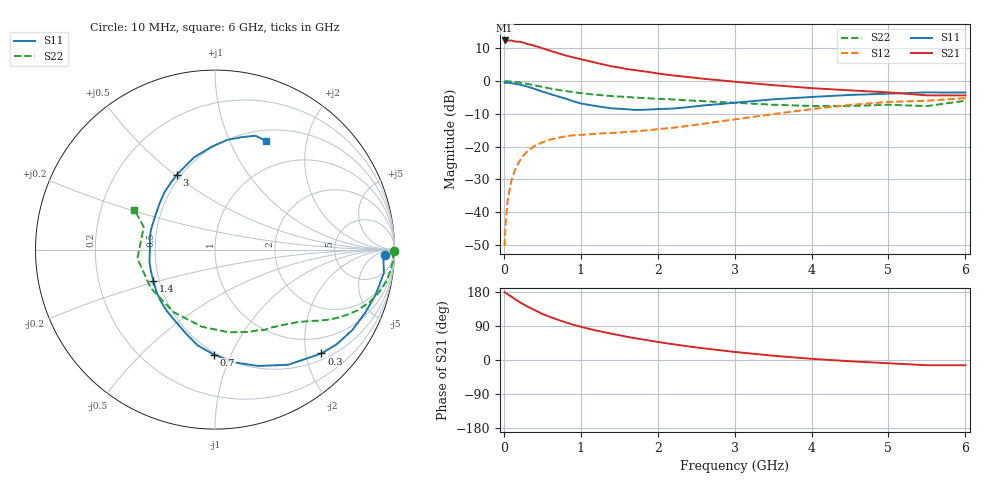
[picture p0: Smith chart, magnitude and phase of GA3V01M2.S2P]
! Infineon Technologies  Discrete & RF Semiconductors
! BF775
! Si NPN RF Bipolar Junction Transistor in SOT23
! VCE = 3 V  IC = 1.2 mA
! Common Emitter S-Parameters:  May  1996
# GHz  S  MA  R  50
!  f  S11  S21  S12  S22
! GHz  MAG  ANG  MAG  ANG  MAG  ANG  MAG  ANG
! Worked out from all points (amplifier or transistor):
!   36 points, 10 MHz to 6 GHz, reference 50 ohm
!   highest |S21| = 12.4 dB at 10 MHz (marker M1)
!   |S21| within 3 dB of that: start of sweep to 583.7 MHz
!   unconditionally stable (mu >= 1): 1.352 GHz to 4.182 GHz; 5.091 GHz to end of sweep
!   at 250 MHz: K = 0.22, MSG = 17.3 dB, |S12| = -22.9 dB
!   at 1.4 GHz: K = 1.03, MAG = 9.1 dB, |S12| = -15.8 dB
!   at 6 GHz: K = 1.03, MAG = -0.6 dB, |S12| = -5.2 dB
!   S11 on the Smith chart (normalised r, x): 10 MHz: 29, -16; 300 MHz: 0.63, -2.31; 700 MHz: 0.49, -0.86; 1.4 GHz: 0.46, -0.19; 3 GHz: 0.47, +0.51; 6 GHz: 0.63, +1.38
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0.01  0.9483 -1.7  4.187 179.0  0.003 90.8  0.9997 -0.6
0.02  0.94 -3.2  4.084 177.3  0.006 89.2  0.9915 -1.3
0.05  0.9499 -7.9  4.169 173.4  0.0154 84.7  0.9948 -3.4
0.1  0.9292 -15.8  4.179 167.1  0.0308 80.8  0.9832 -6.8
0.15  0.9071 -23.0  4.025 159.8  0.0456 75.9  0.9734 -10.1
0.2  0.887 -30.3  4.009 153.7  0.0591 71.6  0.9546 -13.1
0.25  0.8595 -37.8  3.896 147.5  0.072 67.1  0.9334 -16.1
0.3  0.8286 -44.3  3.709 141.9  0.0832 63.6  0.9105 -18.6
0.4  0.7606 -57.5  3.477 131.8  0.1023 57.1  0.8645 -23.0
0.5  0.6918 -69.6  3.185 121.6  0.1161 51.5  0.8144 -26.7
0.7  0.585 -90.6  2.687 106.4  0.1358 43.7  0.7386 -32.0
0.9  0.4934 -109.4  2.311 93.2  0.1485 38.7  0.6805 -35.7
1.1  0.435 -128.1  2.036 82.7  0.154 36.5  0.6357 -39.1
1.4  0.384 -153.3  1.686 69.3  0.1615 35.1  0.5932 -43.8
1.8  0.3638 175.2  1.422 54.4  0.1748 37.3  0.5531 -50.1
2.2  0.3813 151.6  1.219 41.6  0.194 40.0  0.5253 -58.3
3  0.4678 117.2  0.98 21.3  0.2599 42.3  0.4672 -80.5
3.5  0.5268 102.8  0.869 11.3  0.3135 39.8  0.4361 -99.6
4.5  0.6147 83.7  0.723 -3.3  0.4324 28.4  0.4168 -148.9
5  0.6437 76.7  0.673 -8.6  0.4811 20.5  0.4353 -173.4
5.5  0.6735 70.4  0.606 -13.8  0.501 11.7  0.4162 162.5
6  0.6687 64.7  0.605 -13.8  0.5501 7.1  0.5009 153.7
